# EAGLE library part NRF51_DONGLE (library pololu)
https://www.nordicsemi.com/eng/Products/nRF51-Dongle The nRF51 Dongle is a low-cost, versatile USB development dongle for Bluetooth® Smart, ANT and 2.4GHz proprietary applications using the nRF51 Series SoC. The dongle supports development for nRF51822 and nRF51422 SoCs.
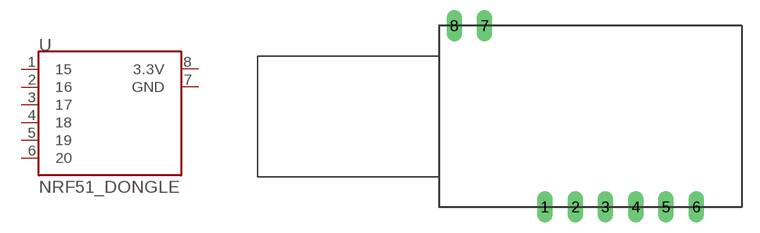
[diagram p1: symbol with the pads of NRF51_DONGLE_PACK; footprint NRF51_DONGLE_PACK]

Designator prefix -

## NRF51_DONGLE  [NRF51_DONGLE_PACK]
1  15
2  16
3  17
4  18
5  19
6  20
7  GND  pwr
8  3.3V  pwr

## Footprint NRF51_DONGLE_PACK (pad centres in mm)
Dual In Line Package
drill 0.813 long: 1 0,0; 2 2.54,0; 3 5.08,0; 4 7.62,0; 5 10.16,0; 6 12.7,0; 7 -5.08,15.24; 8 -7.62,15.24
